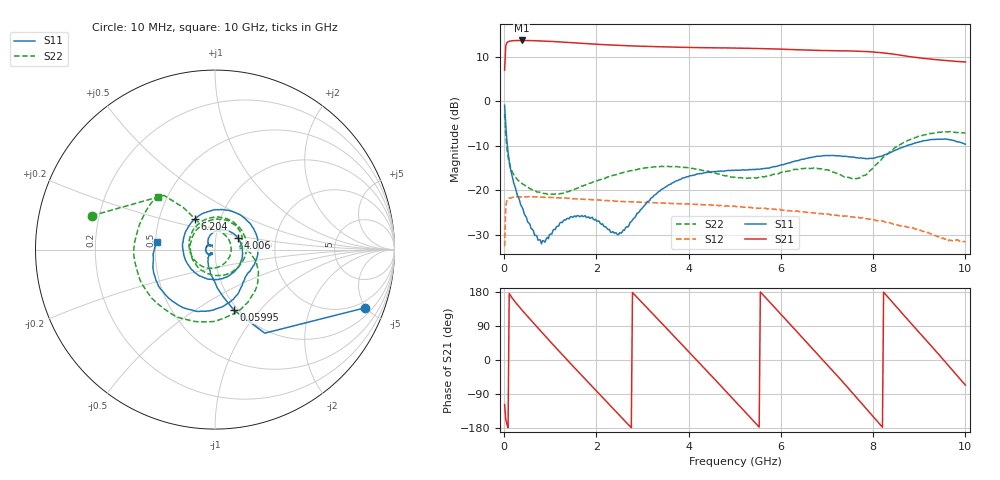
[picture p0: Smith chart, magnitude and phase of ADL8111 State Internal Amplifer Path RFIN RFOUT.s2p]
! Analog Devices Inc.
! Device:  ADL8111
! Description: Bypass Amplifier
! Frequency:  0.00 -  8.00 GHz
! Package:28-Lead Lead Frame Chip Scale Package[LFCSP] 6mm by 6mm
! Conditions:	Vdd = 5.0 V
!		State: Internal Amplifier
!		Path:  RFIN (Port 1) to RFOUT (Port 2)
!		Idq = 70mA
!		Pin = -10 dBm
!		Temp = +25 C (baseplate temperature)
! Freq(Hz)	S11a(dB)	S11p(deg)	S21a(dB)	S21p(deg)	S12a(dB)	S12p(deg)	S22a(dB)	S22p(deg)
# Hz S  dB  R 50
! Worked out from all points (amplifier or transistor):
!   401 points, 10 MHz to 10 GHz, reference 50 ohm
!   highest |S21| = 13.6 dB at 384.6 MHz (marker M1)
!   |S21| within 3 dB of that: 26.69 MHz to 8.395 GHz (8.368 GHz wide, 199 % of centre)
!   unconditionally stable (mu >= 1): start of sweep to end of sweep
!   at 1.658 GHz: K = 1.57, MAG = 13.1 dB, |S12| = -22.0 dB
!   at 5.005 GHz: K = 1.99, MAG = 12.1 dB, |S12| = -23.6 dB
!   at 10 GHz: K = 5.23, MAG = 10.1 dB, |S12| = -31.7 dB
!   S11 on the Smith chart (normalised r, x): 10 MHz: 1.48, -4.92; 59.95 MHz: 0.96, -0.74; 4.006 GHz: 1.28, +0.17; 6.204 GHz: 0.76, +0.27; 10 GHz: 0.51, +0.05
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1e7  -0.94 -21.2  6.95 -117.3  -32.60 115.7  -2.96 164.6
5.995e7  -9.05 -72.7  13.09 -170.2  -22.36 22.4  -10.63 127.0
3.84625e8  -23.74 -125.6  13.61 132.0  -21.49 -41.1  -18.55 95.1
7.34275e8  -31.26 -141.1  13.54 84.2  -21.59 -85.9  -20.45 42.0
1.133875e9  -28.23 -130.2  13.32 30.8  -21.73 -135.5  -20.86 -26.3
1.683325e9  -25.71 174.0  12.97 -41.0  -22.02 157.1  -19.10 -110.8
2.132875e9  -27.59 140.1  12.69 -99.0  -22.25 103.6  -17.44 -164.0
2.632375e9  -28.45 142.9  12.43 -162.8  -22.61 43.6  -15.95 145.0
3.35665e9  -20.34 95.0  12.20 104.6  -22.89 -43.5  -14.78 74.3
4.006e9  -16.88 26.2  12.04 21.2  -23.12 -122.8  -15.02 8.7
4.430575e9  -16.00 -19.9  11.96 -33.5  -23.27 -175.1  -15.75 -39.4
5.005e9  -15.52 -83.6  11.89 -108.3  -23.61 113.6  -17.14 -113.8
5.579425e9  -15.24 -154.4  11.77 176.3  -24.07 41.1  -17.02 168.7
6.2038e9  -13.85 123.5  11.57 93.7  -24.67 -37.6  -15.65 98.8
6.678325e9  -12.63 64.6  11.40 30.8  -25.11 -97.5  -15.12 53.9
7.077925e9  -12.21 20.9  11.30 -22.2  -25.61 -148.6  -15.80 22.7
7.55245e9  -12.59 -19.0  11.24 -86.7  -26.05 150.8  -17.41 3.8
8.002e9  -12.86 -41.8  11.02 -149.2  -26.66 91.8  -14.96 -1.7
8.35165e9  -11.69 -57.0  10.64 161.6  -27.31 45.8  -11.48 -25.3
8.976025e9  -9.25 -96.9  9.73 75.7  -28.82 -35.0  -7.95 -91.1
9.475525e9  -8.56 -138.0  9.19 7.5  -30.63 -97.9  -6.99 -152.1
1e10  -9.70 172.9  8.78 -66.5  -31.67 -159.1  -7.23 137.2
